(* Logix 5000 AddOnInstructionDefinition export HI6200_Faceplate_IT_AOI; software revision 30.00; part 2 of 2 *)
(* tags used below, declared in another part *)
   Inp_hi6200 : _0102:Hardy6200Series_F6857DC7:I:0;
   Out_hi6200 : _0102:Hardy6200Series_52E4DDE0:O:0;
   IT_Status : DINT;   // Integrated Technician status indication
   pm_49C1 : REAL;   // WAVERSAVER VAR ch 1
   pm_49C2 : REAL;   // WAVERSAVER VAR ch 2
   pm_49C3 : REAL;   // WAVERSAVER VAR ch 3
   pm_49C8 : REAL;   // WAVERSAVER VAR ref 1
   pm_49C4 : REAL;   // WAVERSAVER VAR ch 4
   pm_49C5 : REAL;   // WAVERSAVER VAR ch 5
   pm_49C6 : REAL;   // WAVERSAVER VAR ch 6
   pm_49C7 : REAL;   // WAVERSAVER VAR ch 7
   pm_49C9 : REAL;   // WAVERSAVER VAR ref 2
   pm_49D0 : DINT;   // RAW VAR results ch 0
   pm_49D1 : DINT;   // RAW VAR results ch 1
   pm_49D2 : DINT;   // RAW VAR results ch 2
   pm_49D3 : DINT;   // RAW VAR results ch 3
   pm_49D8 : DINT;   // RAW VAR results ref 1
   pm_49D4 : DINT;   // RAW VAR results ch 4
   pm_49D5 : DINT;   // RAW VAR results ch 5
   pm_49D6 : DINT;   // RAW VAR results ch 6
   pm_49D7 : DINT;   // RAW VAR results ch 7
   pm_49D9 : DINT;   // RAW VAR results ref 2
   pm_49E0 : DINT;   // WAVERSAVER VAR results ch 0
   pm_49E1 : DINT;   // WAVERSAVER VAR results ch 1
   pm_49E2 : DINT;   // WAVERSAVER VAR results ch 2
   pm_49E3 : DINT;   // WAVERSAVER VAR results ch 3
   pm_49E8 : DINT;   // WAVERSAVER VAR results ref 1
   pm_49E4 : DINT;   // WAVERSAVER VAR results ch 4
   pm_49E5 : DINT;   // WAVERSAVER VAR results ch 5
   pm_49E6 : DINT;   // WAVERSAVER VAR results ch 6
   pm_49E7 : DINT;   // WAVERSAVER VAR results ch 7
   pm_49E9 : DINT;   // WAVERSAVER VAR results ref 2
   rd_rtz : INT;   // return to zero status
   pm_49F0 : DINT;   // RTZ ch 0
   pm_49F1 : DINT;   // RTZ ch 1
   pm_49F2 : DINT;   // RTZ ch 2
   pm_49F3 : DINT;   // RTZ ch 3
   pm_49F4 : DINT;   // RTZ ch 4
   pm_49F5 : DINT;   // RTZ ch 5
   pm_49F6 : DINT;   // RTZ ch 6
   pm_49F7 : DINT;   // RTZ ch 7
   pm_498C : DINT;   // RTZ combined
   IT_running_status : DINT;   // running/status indication
   rd_ws_var : INT;   // trigger to read WAVERSAVER variation
   rd_raw_rst : INT;   // trigger to read raw variation results
   rd_ws_rst : INT;   // trigger to read WAVERSAVER results
   rd_jbox_2_too : BOOL;   // Process control bit
   delay_clear : TIMER;   // time delay to copy value
   read_delay_29 : TIMER;   // time delay to copy value
   read_delay_30 : TIMER;   // time delay to copy value
   read_delay_31 : TIMER;   // time delay to copy value
   read_delay_32 : TIMER;   // time delay to copy value
   read_delay_33 : TIMER;   // time delay to copy value
   read_delay_34 : TIMER;   // time delay to copy value
   read_delay_35 : TIMER;   // time delay to copy value
   read_delay_36 : TIMER;   // time delay to copy value
   read_delay_37 : TIMER;   // time delay to copy value
   read_delay_38 : TIMER;   // time delay to copy value
   read_delay_39 : TIMER;   // time delay to copy value
   read_delay_40 : TIMER;   // time delay to copy value
   read_delay_41 : TIMER;   // time delay to copy value
   read_delay_42 : TIMER;   // time delay to copy value
   read_delay_43 : TIMER;   // time delay to copy value
   read_delay_44 : TIMER;   // time delay to copy value
   read_delay_45 : TIMER;   // time delay to copy value
   read_delay_46 : TIMER;   // time delay to copy value
   read_delay_47 : TIMER;   // time delay to copy value
   read_delay_48 : TIMER;   // time delay to copy value
   read_delay_49 : TIMER;   // time delay to copy value
   read_delay_50 : TIMER;   // time delay to copy value
   read_delay_51 : TIMER;   // time delay to copy value
   read_delay_52 : TIMER;   // time delay to copy value
   read_delay_53 : TIMER;   // time delay to copy value
   read_delay_54 : TIMER;   // time delay to copy value
   read_delay_55 : TIMER;   // time delay to copy value
   read_delay_56 : TIMER;   // time delay to copy value
   read_delay_57 : TIMER;   // time delay to copy value
   read_delay_58 : TIMER;   // time delay to copy value
   read_delay_59 : TIMER;   // time delay to copy value
   read_delay_60 : TIMER;   // time delay to copy value
   read_delay_61 : TIMER;   // time delay to copy value
   read_delay_62 : TIMER;   // time delay to copy value
   read_delay_63 : TIMER;   // time delay to copy value
   read_delay_64 : TIMER;   // time delay to copy value
   read_delay_65 : TIMER;   // time delay to copy value
   read_delay_66 : TIMER;   // time delay to copy value
   read_delay_67 : TIMER;   // time delay to copy value
   clear_status : BOOL;   // process control bit
(* HI6200_Faceplate_IT_AOI, continued *)

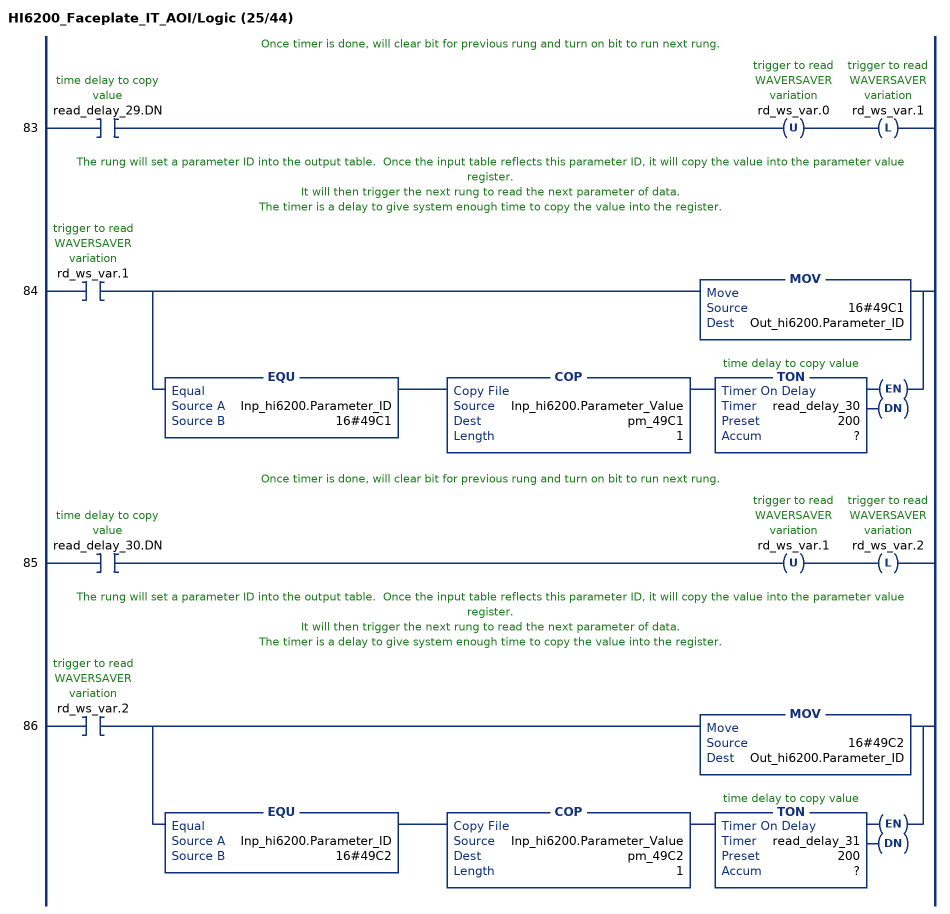
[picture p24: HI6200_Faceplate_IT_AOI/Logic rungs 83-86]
   // Once timer is done, will clear bit for previous rung and turn on bit to run next rung.
   83: XIC(read_delay_29.DN)OTU(rd_ws_var.0)OTL(rd_ws_var.1);
   // The rung will set a parameter ID into the output table.  Once the input table reflects this parameter ID, it will copy the value into the parameter value register.
   // It will then trigger the next rung to read the next parameter of data.
   // The timer is a delay to give system enough time to copy the value into the register.
   84: XIC(rd_ws_var.1)[MOV(16#49C1,Out_hi6200.Parameter_ID) ,EQU(Inp_hi6200.Parameter_ID,16#49C1) COP(Inp_hi6200.Parameter_Value,pm_49C1,1) TON(read_delay_30,?,?) ];
   // Once timer is done, will clear bit for previous rung and turn on bit to run next rung.
   85: XIC(read_delay_30.DN)OTU(rd_ws_var.1)OTL(rd_ws_var.2);
   // The rung will set a parameter ID into the output table.  Once the input table reflects this parameter ID, it will copy the value into the parameter value register.
   // It will then trigger the next rung to read the next parameter of data.
   // The timer is a delay to give system enough time to copy the value into the register.
   86: XIC(rd_ws_var.2)[MOV(16#49C2,Out_hi6200.Parameter_ID) ,EQU(Inp_hi6200.Parameter_ID,16#49C2) COP(Inp_hi6200.Parameter_Value,pm_49C2,1) TON(read_delay_31,?,?) ];
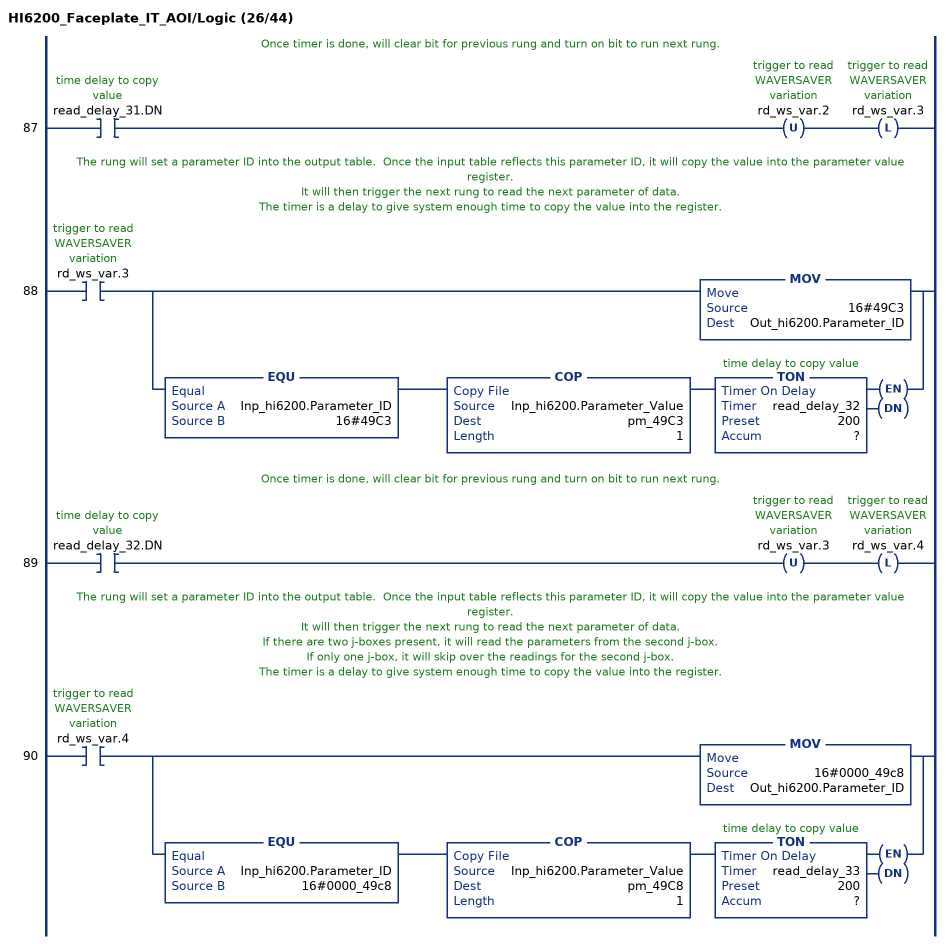
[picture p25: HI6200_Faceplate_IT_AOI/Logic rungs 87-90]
   // Once timer is done, will clear bit for previous rung and turn on bit to run next rung.
   87: XIC(read_delay_31.DN)OTU(rd_ws_var.2)OTL(rd_ws_var.3);
   // The rung will set a parameter ID into the output table.  Once the input table reflects this parameter ID, it will copy the value into the parameter value register.
   // It will then trigger the next rung to read the next parameter of data.
   // The timer is a delay to give system enough time to copy the value into the register.
   88: XIC(rd_ws_var.3)[MOV(16#49C3,Out_hi6200.Parameter_ID) ,EQU(Inp_hi6200.Parameter_ID,16#49C3) COP(Inp_hi6200.Parameter_Value,pm_49C3,1) TON(read_delay_32,?,?) ];
   // Once timer is done, will clear bit for previous rung and turn on bit to run next rung.
   89: XIC(read_delay_32.DN)OTU(rd_ws_var.3)OTL(rd_ws_var.4);
   // The rung will set a parameter ID into the output table.  Once the input table reflects this parameter ID, it will copy the value into the parameter value register.
   // It will then trigger the next rung to read the next parameter of data.
   // If there are two j-boxes present, it will read the parameters from the second j-box.
   // If only one j-box, it will skip over the readings for the second j-box.
   // The timer is a delay to give system enough time to copy the value into the register.
   90: XIC(rd_ws_var.4)[MOV(16#0000_49c8,Out_hi6200.Parameter_ID) ,EQU(Inp_hi6200.Parameter_ID,16#0000_49c8) COP(Inp_hi6200.Parameter_Value,pm_49C8,1) TON(read_delay_33,?,?) ];
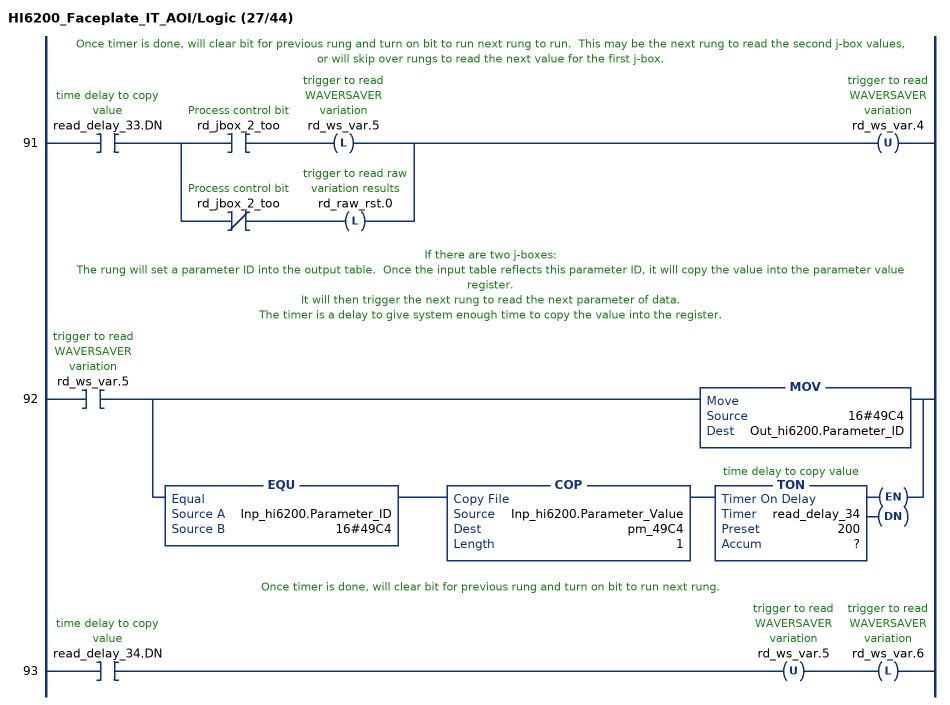
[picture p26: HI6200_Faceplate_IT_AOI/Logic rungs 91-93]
   // Once timer is done, will clear bit for previous rung and turn on bit to run next rung to run.  This may be the next rung to read the second j-box values, or will skip over rungs to read the next value for the first j-box.
   91: XIC(read_delay_33.DN)[XIC(rd_jbox_2_too) OTL(rd_ws_var.5) ,XIO(rd_jbox_2_too) OTL(rd_raw_rst.0) ]OTU(rd_ws_var.4);
   // If there are two j-boxes:
   // The rung will set a parameter ID into the output table.  Once the input table reflects this parameter ID, it will copy the value into the parameter value register.
   // It will then trigger the next rung to read the next parameter of data.
   // The timer is a delay to give system enough time to copy the value into the register.
   92: XIC(rd_ws_var.5)[MOV(16#49C4,Out_hi6200.Parameter_ID) ,EQU(Inp_hi6200.Parameter_ID,16#49C4) COP(Inp_hi6200.Parameter_Value,pm_49C4,1) TON(read_delay_34,?,?) ];
   // Once timer is done, will clear bit for previous rung and turn on bit to run next rung.
   93: XIC(read_delay_34.DN)OTU(rd_ws_var.5)OTL(rd_ws_var.6);
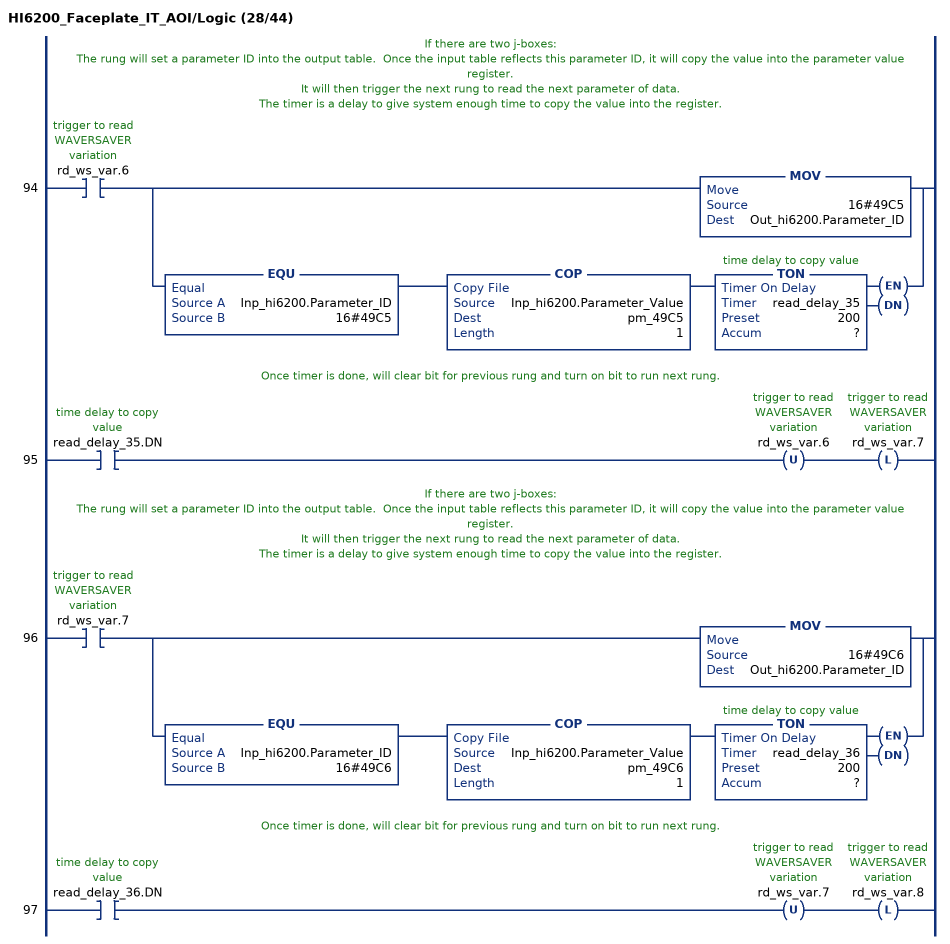
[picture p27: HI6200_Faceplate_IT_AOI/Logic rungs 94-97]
   // If there are two j-boxes:
   // The rung will set a parameter ID into the output table.  Once the input table reflects this parameter ID, it will copy the value into the parameter value register.
   // It will then trigger the next rung to read the next parameter of data.
   // The timer is a delay to give system enough time to copy the value into the register.
   94: XIC(rd_ws_var.6)[MOV(16#49C5,Out_hi6200.Parameter_ID) ,EQU(Inp_hi6200.Parameter_ID,16#49C5) COP(Inp_hi6200.Parameter_Value,pm_49C5,1) TON(read_delay_35,?,?) ];
   // Once timer is done, will clear bit for previous rung and turn on bit to run next rung.
   95: XIC(read_delay_35.DN)OTU(rd_ws_var.6)OTL(rd_ws_var.7);
   // If there are two j-boxes:
   // The rung will set a parameter ID into the output table.  Once the input table reflects this parameter ID, it will copy the value into the parameter value register.
   // It will then trigger the next rung to read the next parameter of data.
   // The timer is a delay to give system enough time to copy the value into the register.
   96: XIC(rd_ws_var.7)[MOV(16#49C6,Out_hi6200.Parameter_ID) ,EQU(Inp_hi6200.Parameter_ID,16#49C6) COP(Inp_hi6200.Parameter_Value,pm_49C6,1) TON(read_delay_36,?,?) ];
   // Once timer is done, will clear bit for previous rung and turn on bit to run next rung.
   97: XIC(read_delay_36.DN)OTU(rd_ws_var.7)OTL(rd_ws_var.8);
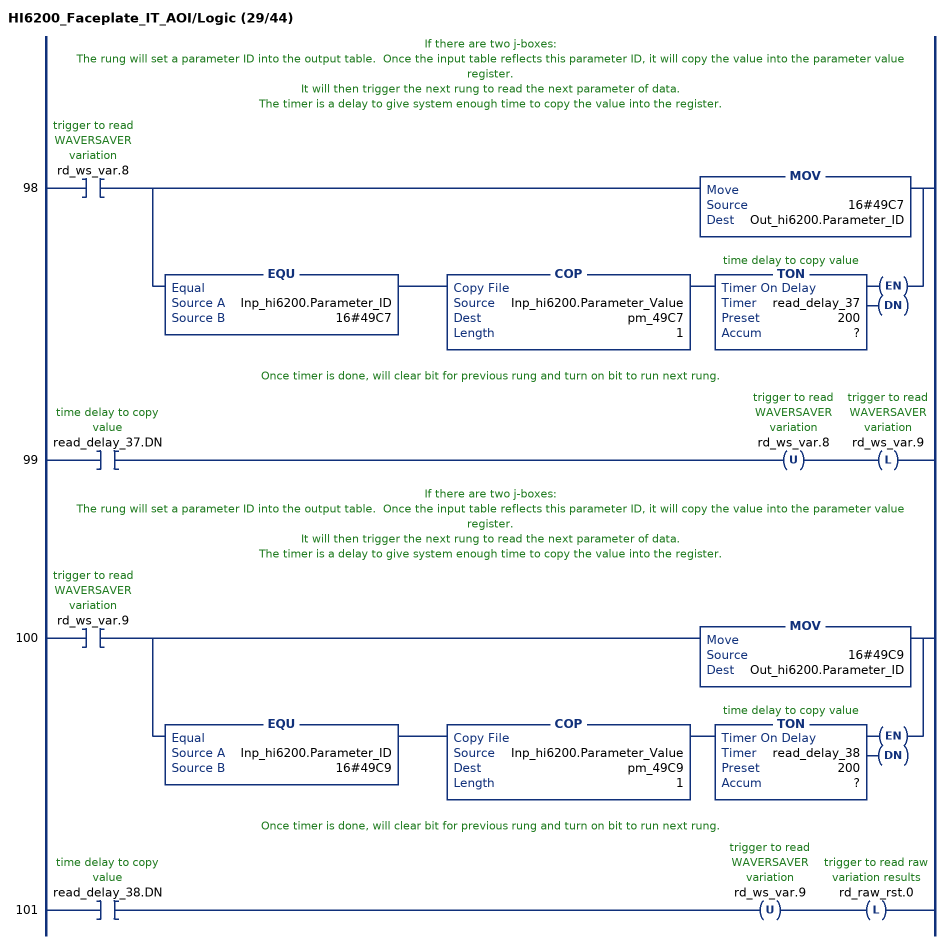
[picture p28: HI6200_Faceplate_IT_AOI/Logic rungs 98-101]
   // If there are two j-boxes:
   // The rung will set a parameter ID into the output table.  Once the input table reflects this parameter ID, it will copy the value into the parameter value register.
   // It will then trigger the next rung to read the next parameter of data.
   // The timer is a delay to give system enough time to copy the value into the register.
   98: XIC(rd_ws_var.8)[MOV(16#49C7,Out_hi6200.Parameter_ID) ,EQU(Inp_hi6200.Parameter_ID,16#49C7) COP(Inp_hi6200.Parameter_Value,pm_49C7,1) TON(read_delay_37,?,?) ];
   // Once timer is done, will clear bit for previous rung and turn on bit to run next rung.
   99: XIC(read_delay_37.DN)OTU(rd_ws_var.8)OTL(rd_ws_var.9);
   // If there are two j-boxes:
   // The rung will set a parameter ID into the output table.  Once the input table reflects this parameter ID, it will copy the value into the parameter value register.
   // It will then trigger the next rung to read the next parameter of data.
   // The timer is a delay to give system enough time to copy the value into the register.
   100: XIC(rd_ws_var.9)[MOV(16#49C9,Out_hi6200.Parameter_ID) ,EQU(Inp_hi6200.Parameter_ID,16#49C9) COP(Inp_hi6200.Parameter_Value,pm_49C9,1) TON(read_delay_38,?,?) ];
   // Once timer is done, will clear bit for previous rung and turn on bit to run next rung.
   101: XIC(read_delay_38.DN)OTU(rd_ws_var.9)OTL(rd_raw_rst.0);
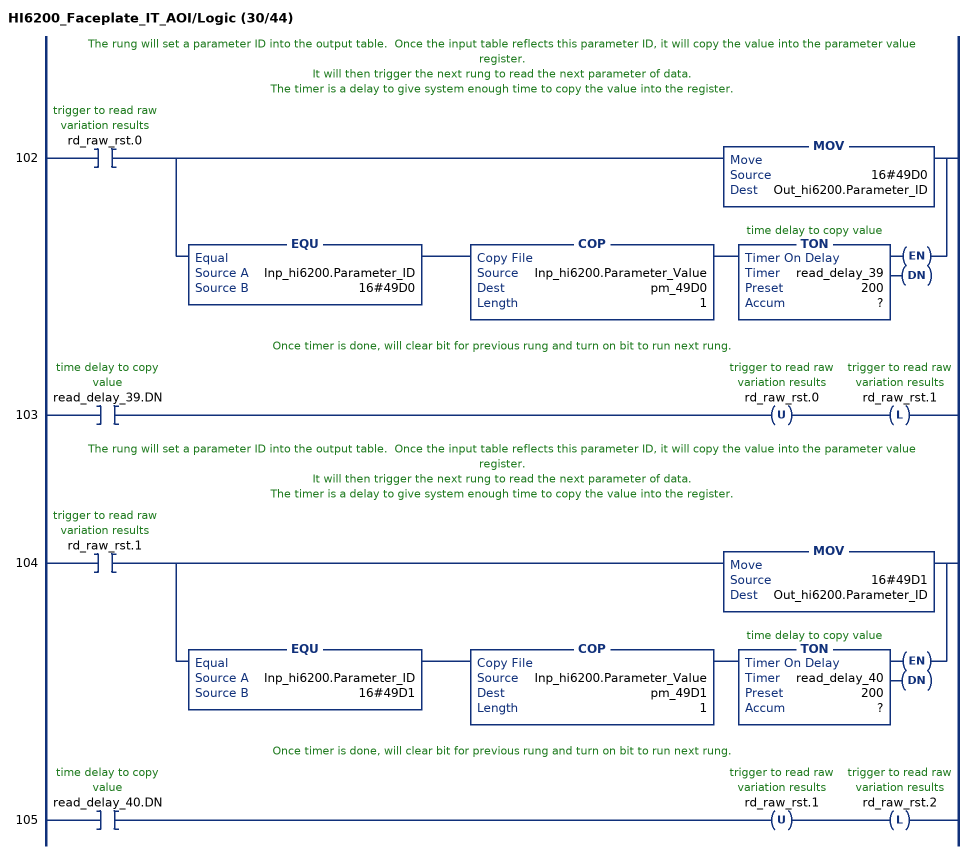
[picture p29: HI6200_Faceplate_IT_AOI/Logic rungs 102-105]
   // The rung will set a parameter ID into the output table.  Once the input table reflects this parameter ID, it will copy the value into the parameter value register.
   // It will then trigger the next rung to read the next parameter of data.
   // The timer is a delay to give system enough time to copy the value into the register.
   102: XIC(rd_raw_rst.0)[MOV(16#49D0,Out_hi6200.Parameter_ID) ,EQU(Inp_hi6200.Parameter_ID,16#49D0) COP(Inp_hi6200.Parameter_Value,pm_49D0,1) TON(read_delay_39,?,?) ];
   // Once timer is done, will clear bit for previous rung and turn on bit to run next rung.
   103: XIC(read_delay_39.DN)OTU(rd_raw_rst.0)OTL(rd_raw_rst.1);
   // The rung will set a parameter ID into the output table.  Once the input table reflects this parameter ID, it will copy the value into the parameter value register.
   // It will then trigger the next rung to read the next parameter of data.
   // The timer is a delay to give system enough time to copy the value into the register.
   104: XIC(rd_raw_rst.1)[MOV(16#49D1,Out_hi6200.Parameter_ID) ,EQU(Inp_hi6200.Parameter_ID,16#49D1) COP(Inp_hi6200.Parameter_Value,pm_49D1,1) TON(read_delay_40,?,?) ];
   // Once timer is done, will clear bit for previous rung and turn on bit to run next rung.
   105: XIC(read_delay_40.DN)OTU(rd_raw_rst.1)OTL(rd_raw_rst.2);
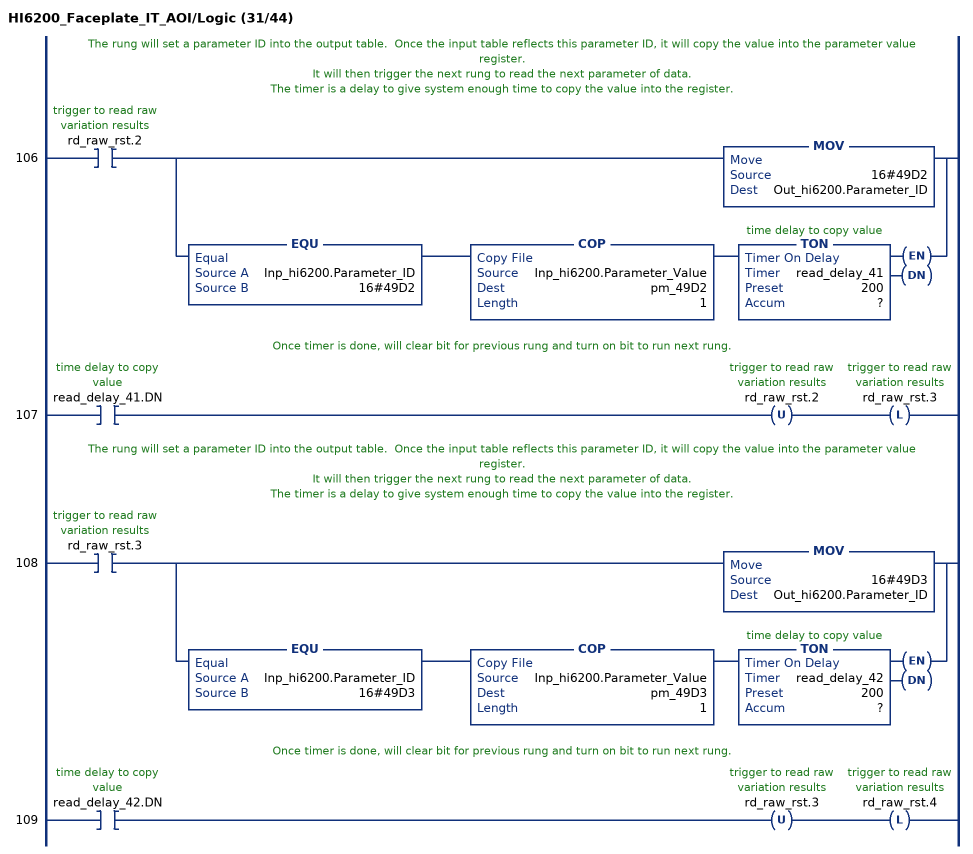
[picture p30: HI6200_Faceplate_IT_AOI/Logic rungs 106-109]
   // The rung will set a parameter ID into the output table.  Once the input table reflects this parameter ID, it will copy the value into the parameter value register.
   // It will then trigger the next rung to read the next parameter of data.
   // The timer is a delay to give system enough time to copy the value into the register.
   106: XIC(rd_raw_rst.2)[MOV(16#49D2,Out_hi6200.Parameter_ID) ,EQU(Inp_hi6200.Parameter_ID,16#49D2) COP(Inp_hi6200.Parameter_Value,pm_49D2,1) TON(read_delay_41,?,?) ];
   // Once timer is done, will clear bit for previous rung and turn on bit to run next rung.
   107: XIC(read_delay_41.DN)OTU(rd_raw_rst.2)OTL(rd_raw_rst.3);
   // The rung will set a parameter ID into the output table.  Once the input table reflects this parameter ID, it will copy the value into the parameter value register.
   // It will then trigger the next rung to read the next parameter of data.
   // The timer is a delay to give system enough time to copy the value into the register.
   108: XIC(rd_raw_rst.3)[MOV(16#49D3,Out_hi6200.Parameter_ID) ,EQU(Inp_hi6200.Parameter_ID,16#49D3) COP(Inp_hi6200.Parameter_Value,pm_49D3,1) TON(read_delay_42,?,?) ];
   // Once timer is done, will clear bit for previous rung and turn on bit to run next rung.
   109: XIC(read_delay_42.DN)OTU(rd_raw_rst.3)OTL(rd_raw_rst.4);
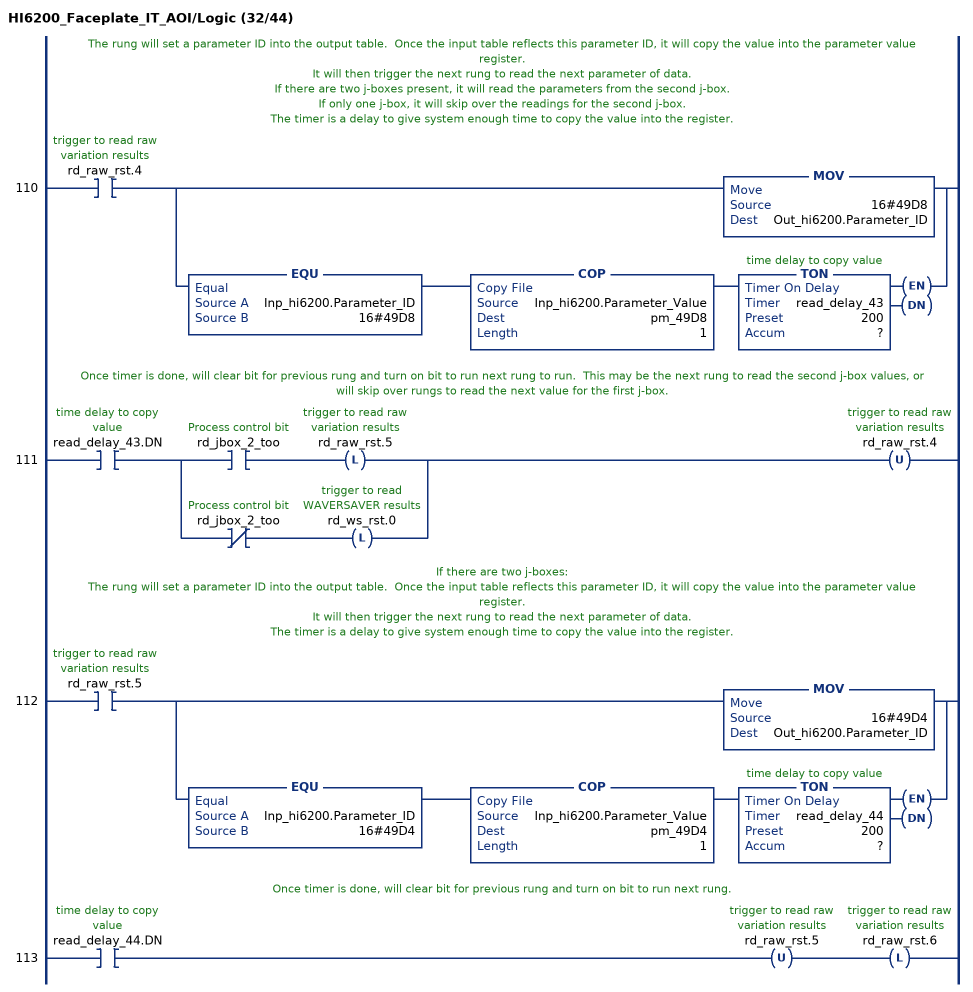
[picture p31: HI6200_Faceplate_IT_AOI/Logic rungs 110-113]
   // The rung will set a parameter ID into the output table.  Once the input table reflects this parameter ID, it will copy the value into the parameter value register.
   // It will then trigger the next rung to read the next parameter of data.
   // If there are two j-boxes present, it will read the parameters from the second j-box.
   // If only one j-box, it will skip over the readings for the second j-box.
   // The timer is a delay to give system enough time to copy the value into the register.
   110: XIC(rd_raw_rst.4)[MOV(16#49D8,Out_hi6200.Parameter_ID) ,EQU(Inp_hi6200.Parameter_ID,16#49D8) COP(Inp_hi6200.Parameter_Value,pm_49D8,1) TON(read_delay_43,?,?) ];
   // Once timer is done, will clear bit for previous rung and turn on bit to run next rung to run.  This may be the next rung to read the second j-box values, or will skip over rungs to read the next value for the first j-box.
   111: XIC(read_delay_43.DN)[XIC(rd_jbox_2_too) OTL(rd_raw_rst.5) ,XIO(rd_jbox_2_too) OTL(rd_ws_rst.0) ]OTU(rd_raw_rst.4);
   // If there are two j-boxes:
   // The rung will set a parameter ID into the output table.  Once the input table reflects this parameter ID, it will copy the value into the parameter value register.
   // It will then trigger the next rung to read the next parameter of data.
   // The timer is a delay to give system enough time to copy the value into the register.
   112: XIC(rd_raw_rst.5)[MOV(16#49D4,Out_hi6200.Parameter_ID) ,EQU(Inp_hi6200.Parameter_ID,16#49D4) COP(Inp_hi6200.Parameter_Value,pm_49D4,1) TON(read_delay_44,?,?) ];
   // Once timer is done, will clear bit for previous rung and turn on bit to run next rung.
   113: XIC(read_delay_44.DN)OTU(rd_raw_rst.5)OTL(rd_raw_rst.6);
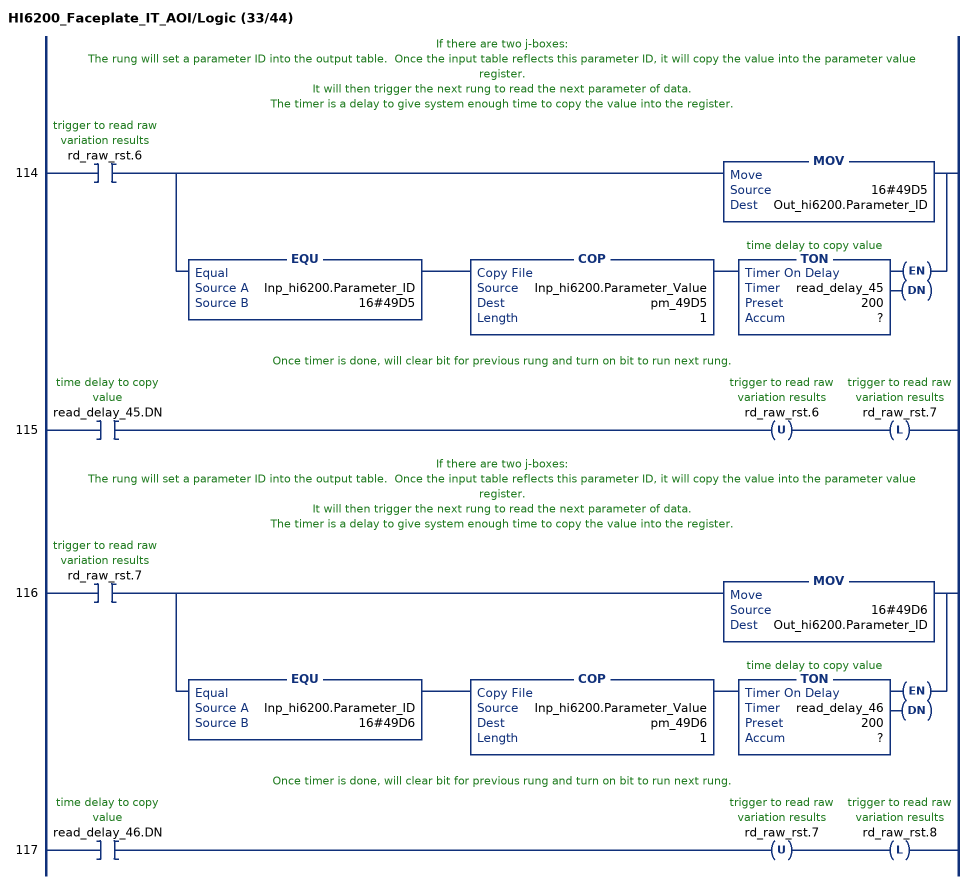
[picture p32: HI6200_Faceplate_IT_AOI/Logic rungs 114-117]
   // If there are two j-boxes:
   // The rung will set a parameter ID into the output table.  Once the input table reflects this parameter ID, it will copy the value into the parameter value register.
   // It will then trigger the next rung to read the next parameter of data.
   // The timer is a delay to give system enough time to copy the value into the register.
   114: XIC(rd_raw_rst.6)[MOV(16#49D5,Out_hi6200.Parameter_ID) ,EQU(Inp_hi6200.Parameter_ID,16#49D5) COP(Inp_hi6200.Parameter_Value,pm_49D5,1) TON(read_delay_45,?,?) ];
   // Once timer is done, will clear bit for previous rung and turn on bit to run next rung.
   115: XIC(read_delay_45.DN)OTU(rd_raw_rst.6)OTL(rd_raw_rst.7);
   // If there are two j-boxes:
   // The rung will set a parameter ID into the output table.  Once the input table reflects this parameter ID, it will copy the value into the parameter value register.
   // It will then trigger the next rung to read the next parameter of data.
   // The timer is a delay to give system enough time to copy the value into the register.
   116: XIC(rd_raw_rst.7)[MOV(16#49D6,Out_hi6200.Parameter_ID) ,EQU(Inp_hi6200.Parameter_ID,16#49D6) COP(Inp_hi6200.Parameter_Value,pm_49D6,1) TON(read_delay_46,?,?) ];
   // Once timer is done, will clear bit for previous rung and turn on bit to run next rung.
   117: XIC(read_delay_46.DN)OTU(rd_raw_rst.7)OTL(rd_raw_rst.8);
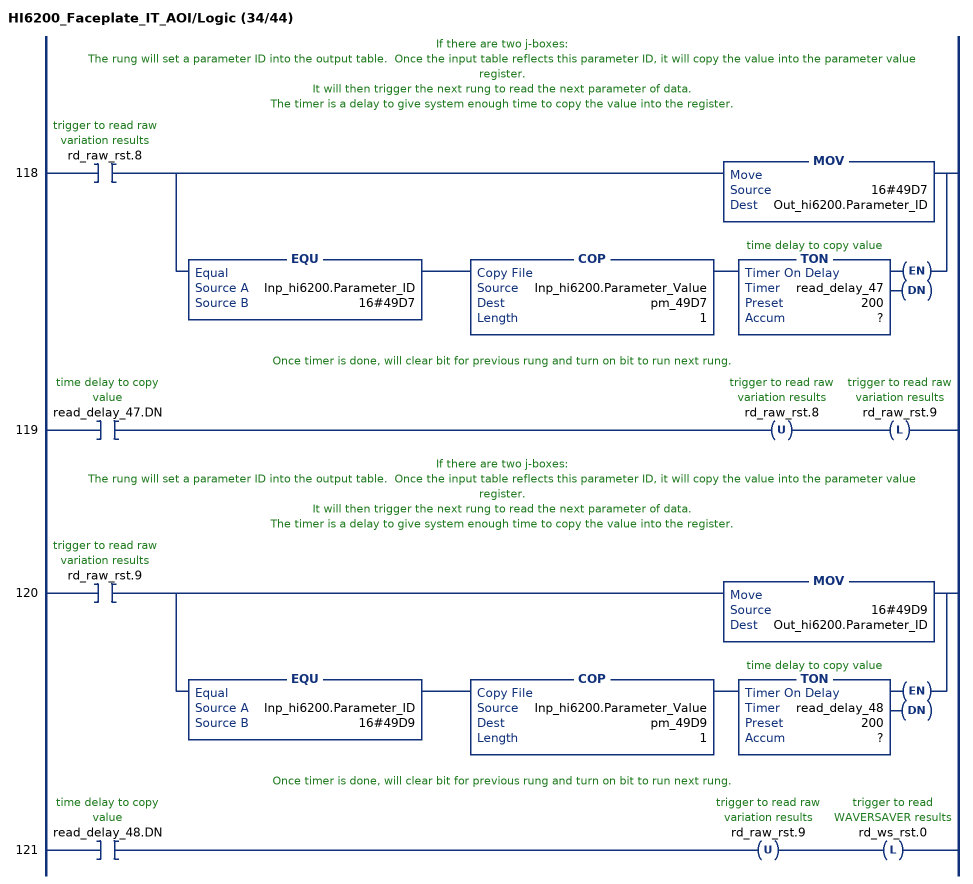
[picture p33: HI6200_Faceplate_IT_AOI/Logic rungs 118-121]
   // If there are two j-boxes:
   // The rung will set a parameter ID into the output table.  Once the input table reflects this parameter ID, it will copy the value into the parameter value register.
   // It will then trigger the next rung to read the next parameter of data.
   // The timer is a delay to give system enough time to copy the value into the register.
   118: XIC(rd_raw_rst.8)[MOV(16#49D7,Out_hi6200.Parameter_ID) ,EQU(Inp_hi6200.Parameter_ID,16#49D7) COP(Inp_hi6200.Parameter_Value,pm_49D7,1) TON(read_delay_47,?,?) ];
   // Once timer is done, will clear bit for previous rung and turn on bit to run next rung.
   119: XIC(read_delay_47.DN)OTU(rd_raw_rst.8)OTL(rd_raw_rst.9);
   // If there are two j-boxes:
   // The rung will set a parameter ID into the output table.  Once the input table reflects this parameter ID, it will copy the value into the parameter value register.
   // It will then trigger the next rung to read the next parameter of data.
   // The timer is a delay to give system enough time to copy the value into the register.
   120: XIC(rd_raw_rst.9)[MOV(16#49D9,Out_hi6200.Parameter_ID) ,EQU(Inp_hi6200.Parameter_ID,16#49D9) COP(Inp_hi6200.Parameter_Value,pm_49D9,1) TON(read_delay_48,?,?) ];
   // Once timer is done, will clear bit for previous rung and turn on bit to run next rung.
   121: XIC(read_delay_48.DN)OTU(rd_raw_rst.9)OTL(rd_ws_rst.0);
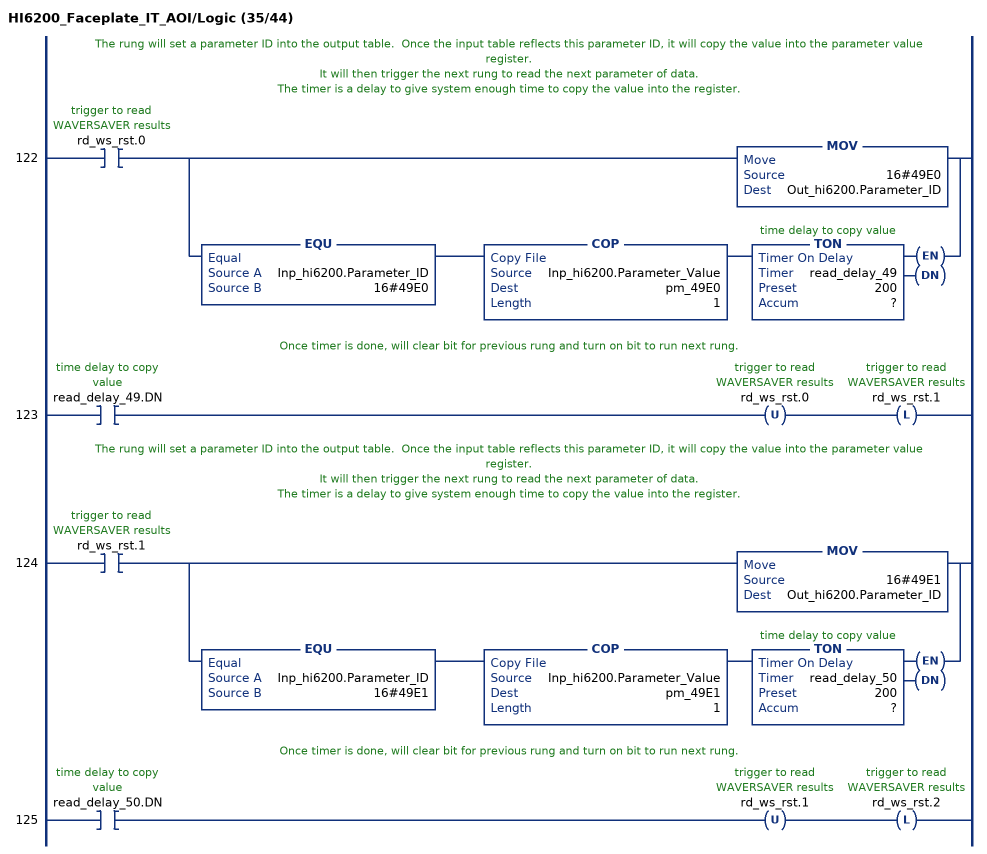
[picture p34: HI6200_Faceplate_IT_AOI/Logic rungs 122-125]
   // The rung will set a parameter ID into the output table.  Once the input table reflects this parameter ID, it will copy the value into the parameter value register.
   // It will then trigger the next rung to read the next parameter of data.
   // The timer is a delay to give system enough time to copy the value into the register.
   122: XIC(rd_ws_rst.0)[MOV(16#49E0,Out_hi6200.Parameter_ID) ,EQU(Inp_hi6200.Parameter_ID,16#49E0) COP(Inp_hi6200.Parameter_Value,pm_49E0,1) TON(read_delay_49,?,?) ];
   // Once timer is done, will clear bit for previous rung and turn on bit to run next rung.
   123: XIC(read_delay_49.DN)OTU(rd_ws_rst.0)OTL(rd_ws_rst.1);
   // The rung will set a parameter ID into the output table.  Once the input table reflects this parameter ID, it will copy the value into the parameter value register.
   // It will then trigger the next rung to read the next parameter of data.
   // The timer is a delay to give system enough time to copy the value into the register.
   124: XIC(rd_ws_rst.1)[MOV(16#49E1,Out_hi6200.Parameter_ID) ,EQU(Inp_hi6200.Parameter_ID,16#49E1) COP(Inp_hi6200.Parameter_Value,pm_49E1,1) TON(read_delay_50,?,?) ];
   // Once timer is done, will clear bit for previous rung and turn on bit to run next rung.
   125: XIC(read_delay_50.DN)OTU(rd_ws_rst.1)OTL(rd_ws_rst.2);
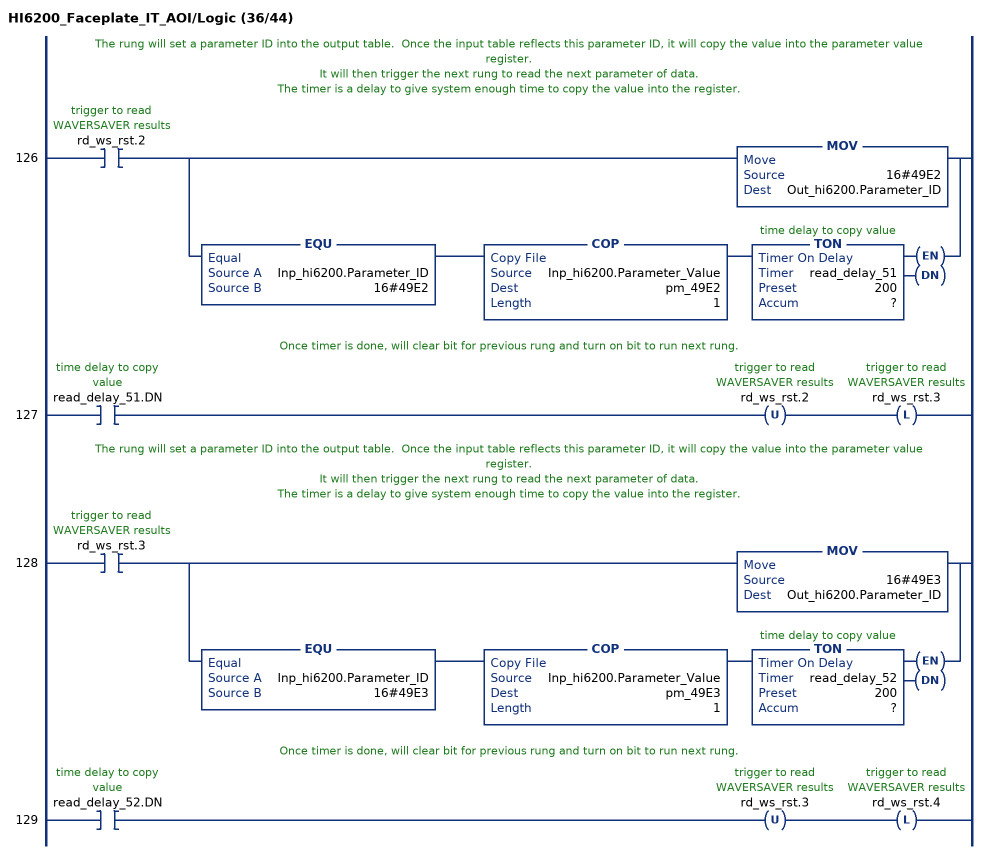
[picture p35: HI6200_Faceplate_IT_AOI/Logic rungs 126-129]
   // The rung will set a parameter ID into the output table.  Once the input table reflects this parameter ID, it will copy the value into the parameter value register.
   // It will then trigger the next rung to read the next parameter of data.
   // The timer is a delay to give system enough time to copy the value into the register.
   126: XIC(rd_ws_rst.2)[MOV(16#49E2,Out_hi6200.Parameter_ID) ,EQU(Inp_hi6200.Parameter_ID,16#49E2) COP(Inp_hi6200.Parameter_Value,pm_49E2,1) TON(read_delay_51,?,?) ];
   // Once timer is done, will clear bit for previous rung and turn on bit to run next rung.
   127: XIC(read_delay_51.DN)OTU(rd_ws_rst.2)OTL(rd_ws_rst.3);
   // The rung will set a parameter ID into the output table.  Once the input table reflects this parameter ID, it will copy the value into the parameter value register.
   // It will then trigger the next rung to read the next parameter of data.
   // The timer is a delay to give system enough time to copy the value into the register.
   128: XIC(rd_ws_rst.3)[MOV(16#49E3,Out_hi6200.Parameter_ID) ,EQU(Inp_hi6200.Parameter_ID,16#49E3) COP(Inp_hi6200.Parameter_Value,pm_49E3,1) TON(read_delay_52,?,?) ];
   // Once timer is done, will clear bit for previous rung and turn on bit to run next rung.
   129: XIC(read_delay_52.DN)OTU(rd_ws_rst.3)OTL(rd_ws_rst.4);
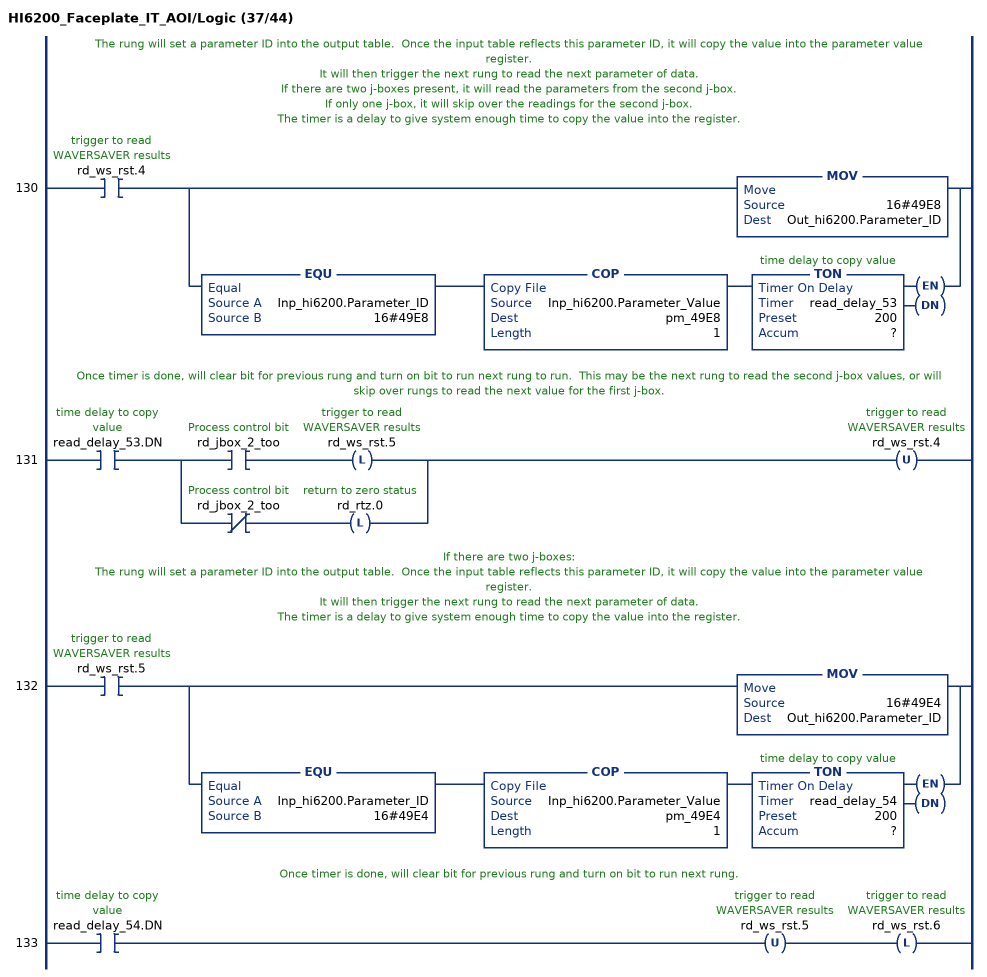
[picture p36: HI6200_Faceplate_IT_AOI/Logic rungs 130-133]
   // The rung will set a parameter ID into the output table.  Once the input table reflects this parameter ID, it will copy the value into the parameter value register.
   // It will then trigger the next rung to read the next parameter of data.
   // If there are two j-boxes present, it will read the parameters from the second j-box.
   // If only one j-box, it will skip over the readings for the second j-box.
   // The timer is a delay to give system enough time to copy the value into the register.
   130: XIC(rd_ws_rst.4)[MOV(16#49E8,Out_hi6200.Parameter_ID) ,EQU(Inp_hi6200.Parameter_ID,16#49E8) COP(Inp_hi6200.Parameter_Value,pm_49E8,1) TON(read_delay_53,?,?) ];
   // Once timer is done, will clear bit for previous rung and turn on bit to run next rung to run.  This may be the next rung to read the second j-box values, or will skip over rungs to read the next value for the first j-box.
   131: XIC(read_delay_53.DN)[XIC(rd_jbox_2_too) OTL(rd_ws_rst.5) ,XIO(rd_jbox_2_too) OTL(rd_rtz.0) ]OTU(rd_ws_rst.4);
   // If there are two j-boxes:
   // The rung will set a parameter ID into the output table.  Once the input table reflects this parameter ID, it will copy the value into the parameter value register.
   // It will then trigger the next rung to read the next parameter of data.
   // The timer is a delay to give system enough time to copy the value into the register.
   132: XIC(rd_ws_rst.5)[MOV(16#49E4,Out_hi6200.Parameter_ID) ,EQU(Inp_hi6200.Parameter_ID,16#49E4) COP(Inp_hi6200.Parameter_Value,pm_49E4,1) TON(read_delay_54,?,?) ];
   // Once timer is done, will clear bit for previous rung and turn on bit to run next rung.
   133: XIC(read_delay_54.DN)OTU(rd_ws_rst.5)OTL(rd_ws_rst.6);
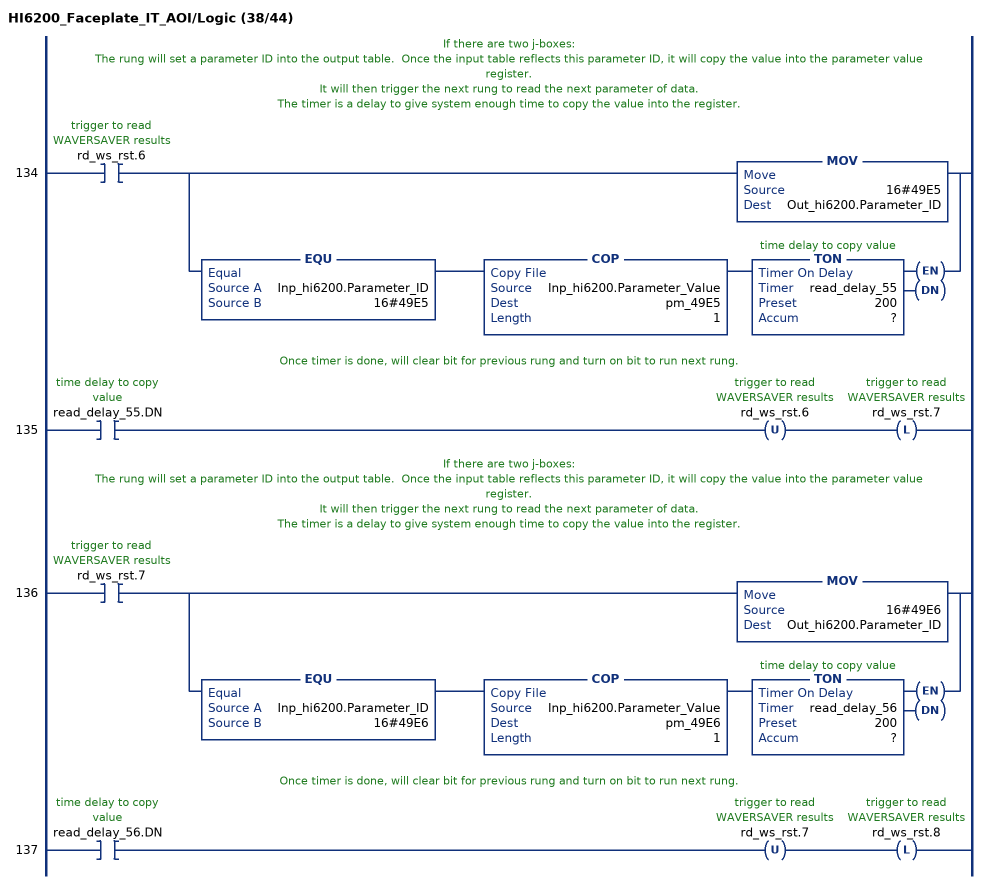
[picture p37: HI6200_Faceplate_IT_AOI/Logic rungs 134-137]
   // If there are two j-boxes:
   // The rung will set a parameter ID into the output table.  Once the input table reflects this parameter ID, it will copy the value into the parameter value register.
   // It will then trigger the next rung to read the next parameter of data.
   // The timer is a delay to give system enough time to copy the value into the register.
   134: XIC(rd_ws_rst.6)[MOV(16#49E5,Out_hi6200.Parameter_ID) ,EQU(Inp_hi6200.Parameter_ID,16#49E5) COP(Inp_hi6200.Parameter_Value,pm_49E5,1) TON(read_delay_55,?,?) ];
   // Once timer is done, will clear bit for previous rung and turn on bit to run next rung.
   135: XIC(read_delay_55.DN)OTU(rd_ws_rst.6)OTL(rd_ws_rst.7);
   // If there are two j-boxes:
   // The rung will set a parameter ID into the output table.  Once the input table reflects this parameter ID, it will copy the value into the parameter value register.
   // It will then trigger the next rung to read the next parameter of data.
   // The timer is a delay to give system enough time to copy the value into the register.
   136: XIC(rd_ws_rst.7)[MOV(16#49E6,Out_hi6200.Parameter_ID) ,EQU(Inp_hi6200.Parameter_ID,16#49E6) COP(Inp_hi6200.Parameter_Value,pm_49E6,1) TON(read_delay_56,?,?) ];
   // Once timer is done, will clear bit for previous rung and turn on bit to run next rung.
   137: XIC(read_delay_56.DN)OTU(rd_ws_rst.7)OTL(rd_ws_rst.8);
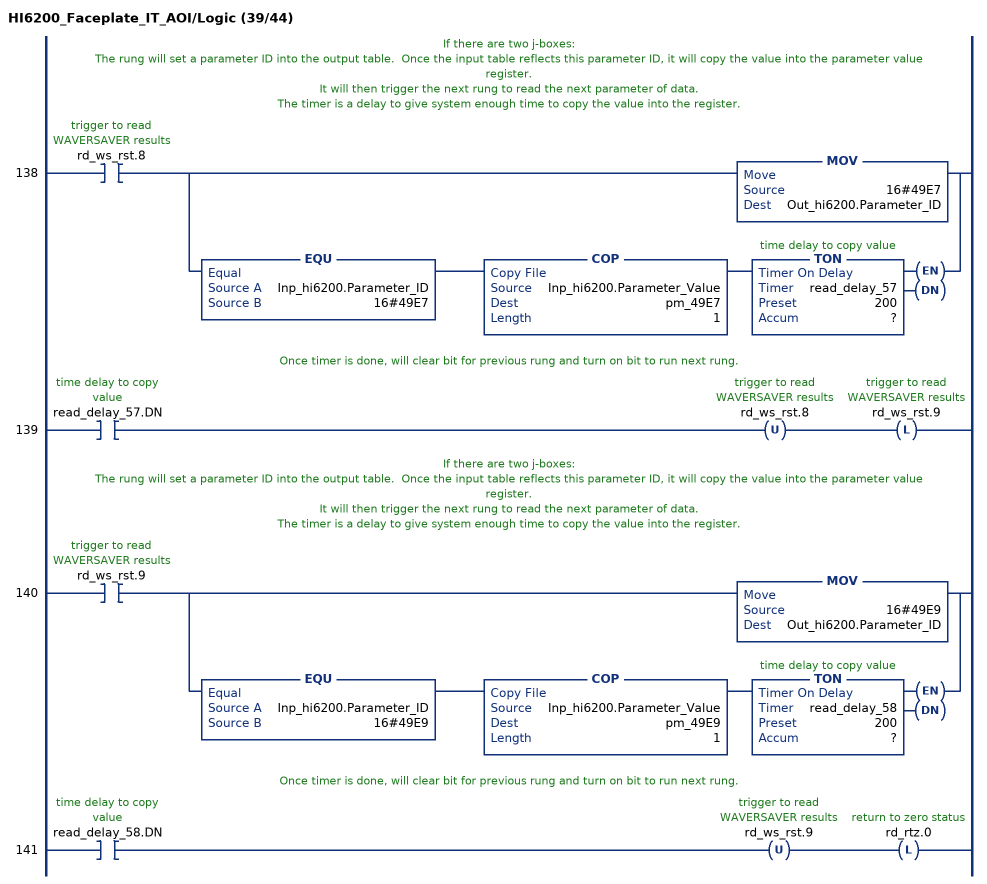
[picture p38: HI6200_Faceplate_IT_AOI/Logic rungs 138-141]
   // If there are two j-boxes:
   // The rung will set a parameter ID into the output table.  Once the input table reflects this parameter ID, it will copy the value into the parameter value register.
   // It will then trigger the next rung to read the next parameter of data.
   // The timer is a delay to give system enough time to copy the value into the register.
   138: XIC(rd_ws_rst.8)[MOV(16#49E7,Out_hi6200.Parameter_ID) ,EQU(Inp_hi6200.Parameter_ID,16#49E7) COP(Inp_hi6200.Parameter_Value,pm_49E7,1) TON(read_delay_57,?,?) ];
   // Once timer is done, will clear bit for previous rung and turn on bit to run next rung.
   139: XIC(read_delay_57.DN)OTU(rd_ws_rst.8)OTL(rd_ws_rst.9);
   // If there are two j-boxes:
   // The rung will set a parameter ID into the output table.  Once the input table reflects this parameter ID, it will copy the value into the parameter value register.
   // It will then trigger the next rung to read the next parameter of data.
   // The timer is a delay to give system enough time to copy the value into the register.
   140: XIC(rd_ws_rst.9)[MOV(16#49E9,Out_hi6200.Parameter_ID) ,EQU(Inp_hi6200.Parameter_ID,16#49E9) COP(Inp_hi6200.Parameter_Value,pm_49E9,1) TON(read_delay_58,?,?) ];
   // Once timer is done, will clear bit for previous rung and turn on bit to run next rung.
   141: XIC(read_delay_58.DN)OTU(rd_ws_rst.9)OTL(rd_rtz.0);
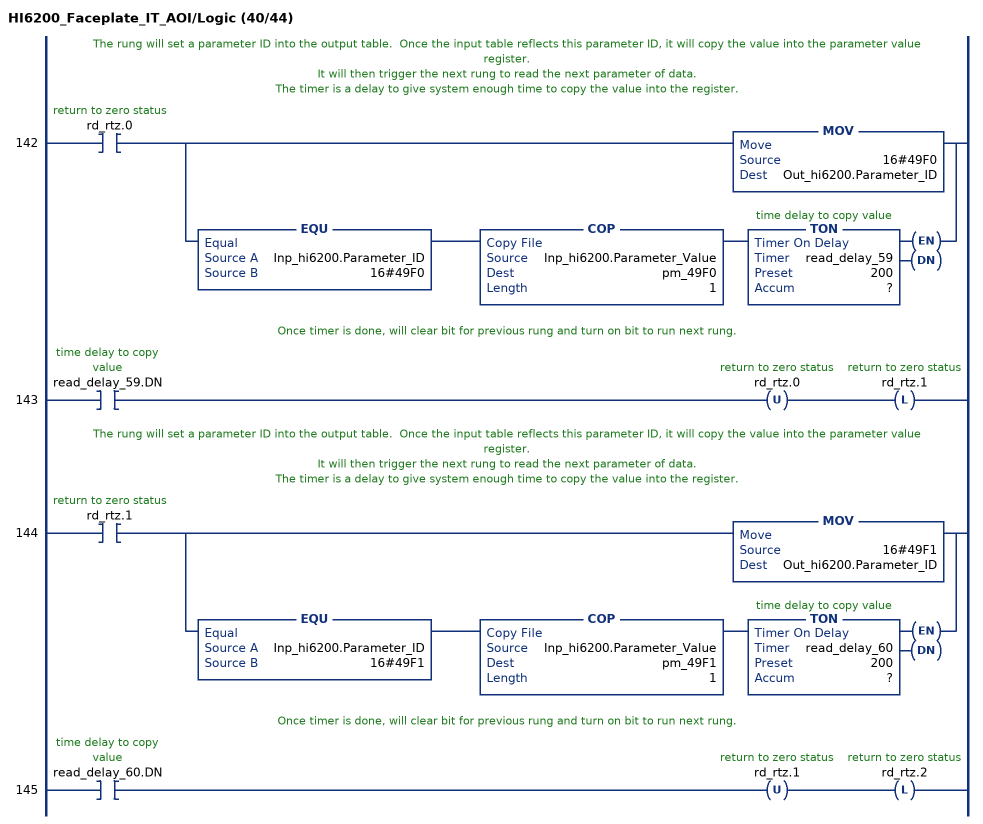
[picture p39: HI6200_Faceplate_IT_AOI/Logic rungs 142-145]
   // The rung will set a parameter ID into the output table.  Once the input table reflects this parameter ID, it will copy the value into the parameter value register.
   // It will then trigger the next rung to read the next parameter of data.
   // The timer is a delay to give system enough time to copy the value into the register.
   142: XIC(rd_rtz.0)[MOV(16#49F0,Out_hi6200.Parameter_ID) ,EQU(Inp_hi6200.Parameter_ID,16#49F0) COP(Inp_hi6200.Parameter_Value,pm_49F0,1) TON(read_delay_59,?,?) ];
   // Once timer is done, will clear bit for previous rung and turn on bit to run next rung.
   143: XIC(read_delay_59.DN)OTU(rd_rtz.0)OTL(rd_rtz.1);
   // The rung will set a parameter ID into the output table.  Once the input table reflects this parameter ID, it will copy the value into the parameter value register.
   // It will then trigger the next rung to read the next parameter of data.
   // The timer is a delay to give system enough time to copy the value into the register.
   144: XIC(rd_rtz.1)[MOV(16#49F1,Out_hi6200.Parameter_ID) ,EQU(Inp_hi6200.Parameter_ID,16#49F1) COP(Inp_hi6200.Parameter_Value,pm_49F1,1) TON(read_delay_60,?,?) ];
   // Once timer is done, will clear bit for previous rung and turn on bit to run next rung.
   145: XIC(read_delay_60.DN)OTU(rd_rtz.1)OTL(rd_rtz.2);
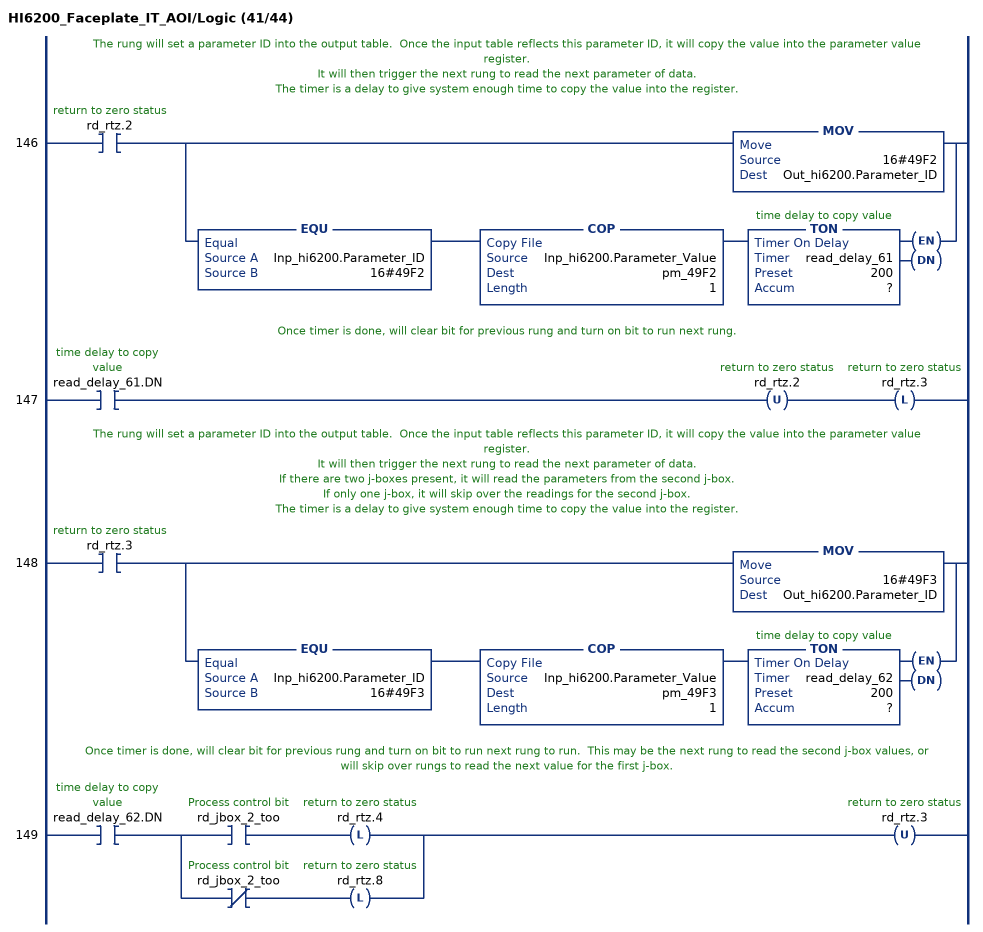
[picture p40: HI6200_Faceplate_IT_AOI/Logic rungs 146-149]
   // The rung will set a parameter ID into the output table.  Once the input table reflects this parameter ID, it will copy the value into the parameter value register.
   // It will then trigger the next rung to read the next parameter of data.
   // The timer is a delay to give system enough time to copy the value into the register.
   146: XIC(rd_rtz.2)[MOV(16#49F2,Out_hi6200.Parameter_ID) ,EQU(Inp_hi6200.Parameter_ID,16#49F2) COP(Inp_hi6200.Parameter_Value,pm_49F2,1) TON(read_delay_61,?,?) ];
   // Once timer is done, will clear bit for previous rung and turn on bit to run next rung.
   147: XIC(read_delay_61.DN)OTU(rd_rtz.2)OTL(rd_rtz.3);
   // The rung will set a parameter ID into the output table.  Once the input table reflects this parameter ID, it will copy the value into the parameter value register.
   // It will then trigger the next rung to read the next parameter of data.
   // If there are two j-boxes present, it will read the parameters from the second j-box.
   // If only one j-box, it will skip over the readings for the second j-box.
   // The timer is a delay to give system enough time to copy the value into the register.
   148: XIC(rd_rtz.3)[MOV(16#49F3,Out_hi6200.Parameter_ID) ,EQU(Inp_hi6200.Parameter_ID,16#49F3) COP(Inp_hi6200.Parameter_Value,pm_49F3,1) TON(read_delay_62,?,?) ];
   // Once timer is done, will clear bit for previous rung and turn on bit to run next rung to run.  This may be the next rung to read the second j-box values, or will skip over rungs to read the next value for the first j-box.
   149: XIC(read_delay_62.DN)[XIC(rd_jbox_2_too) OTL(rd_rtz.4) ,XIO(rd_jbox_2_too) OTL(rd_rtz.8) ]OTU(rd_rtz.3);
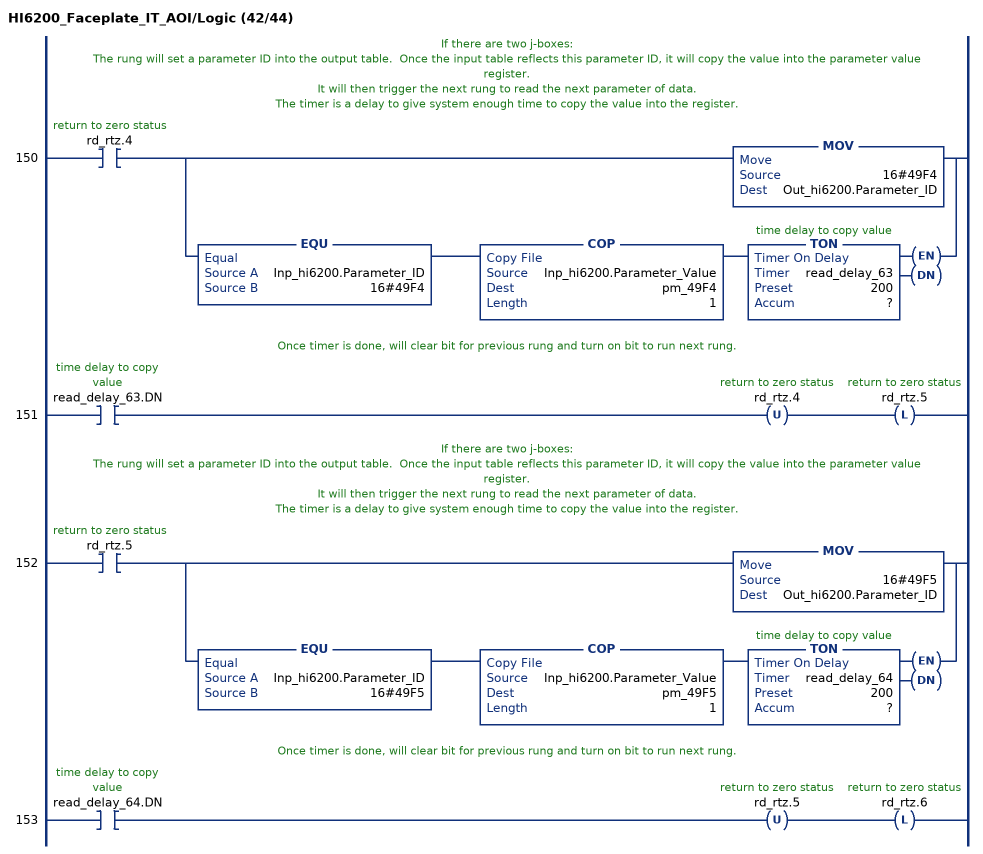
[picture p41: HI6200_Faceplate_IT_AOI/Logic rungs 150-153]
   // If there are two j-boxes:
   // The rung will set a parameter ID into the output table.  Once the input table reflects this parameter ID, it will copy the value into the parameter value register.
   // It will then trigger the next rung to read the next parameter of data.
   // The timer is a delay to give system enough time to copy the value into the register.
   150: XIC(rd_rtz.4)[MOV(16#49F4,Out_hi6200.Parameter_ID) ,EQU(Inp_hi6200.Parameter_ID,16#49F4) COP(Inp_hi6200.Parameter_Value,pm_49F4,1) TON(read_delay_63,?,?) ];
   // Once timer is done, will clear bit for previous rung and turn on bit to run next rung.
   151: XIC(read_delay_63.DN)OTU(rd_rtz.4)OTL(rd_rtz.5);
   // If there are two j-boxes:
   // The rung will set a parameter ID into the output table.  Once the input table reflects this parameter ID, it will copy the value into the parameter value register.
   // It will then trigger the next rung to read the next parameter of data.
   // The timer is a delay to give system enough time to copy the value into the register.
   152: XIC(rd_rtz.5)[MOV(16#49F5,Out_hi6200.Parameter_ID) ,EQU(Inp_hi6200.Parameter_ID,16#49F5) COP(Inp_hi6200.Parameter_Value,pm_49F5,1) TON(read_delay_64,?,?) ];
   // Once timer is done, will clear bit for previous rung and turn on bit to run next rung.
   153: XIC(read_delay_64.DN)OTU(rd_rtz.5)OTL(rd_rtz.6);
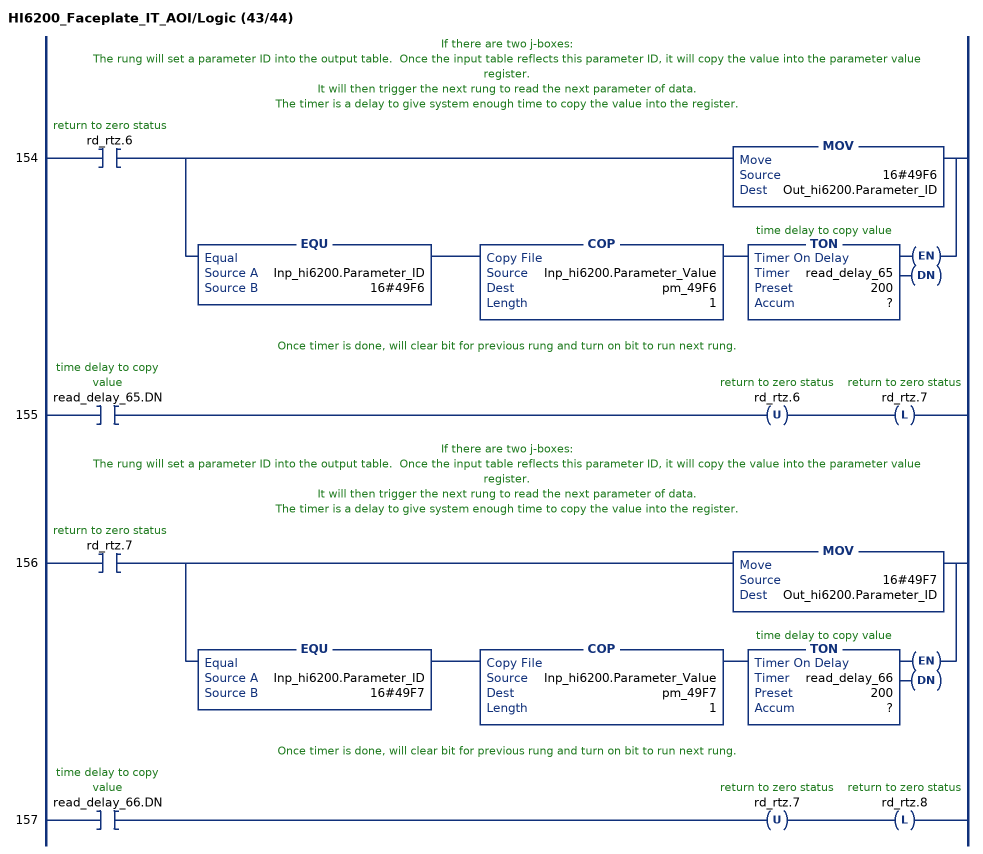
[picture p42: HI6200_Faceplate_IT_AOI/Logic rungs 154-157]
   // If there are two j-boxes:
   // The rung will set a parameter ID into the output table.  Once the input table reflects this parameter ID, it will copy the value into the parameter value register.
   // It will then trigger the next rung to read the next parameter of data.
   // The timer is a delay to give system enough time to copy the value into the register.
   154: XIC(rd_rtz.6)[MOV(16#49F6,Out_hi6200.Parameter_ID) ,EQU(Inp_hi6200.Parameter_ID,16#49F6) COP(Inp_hi6200.Parameter_Value,pm_49F6,1) TON(read_delay_65,?,?) ];
   // Once timer is done, will clear bit for previous rung and turn on bit to run next rung.
   155: XIC(read_delay_65.DN)OTU(rd_rtz.6)OTL(rd_rtz.7);
   // If there are two j-boxes:
   // The rung will set a parameter ID into the output table.  Once the input table reflects this parameter ID, it will copy the value into the parameter value register.
   // It will then trigger the next rung to read the next parameter of data.
   // The timer is a delay to give system enough time to copy the value into the register.
   156: XIC(rd_rtz.7)[MOV(16#49F7,Out_hi6200.Parameter_ID) ,EQU(Inp_hi6200.Parameter_ID,16#49F7) COP(Inp_hi6200.Parameter_Value,pm_49F7,1) TON(read_delay_66,?,?) ];
   // Once timer is done, will clear bit for previous rung and turn on bit to run next rung.
   157: XIC(read_delay_66.DN)OTU(rd_rtz.7)OTL(rd_rtz.8);
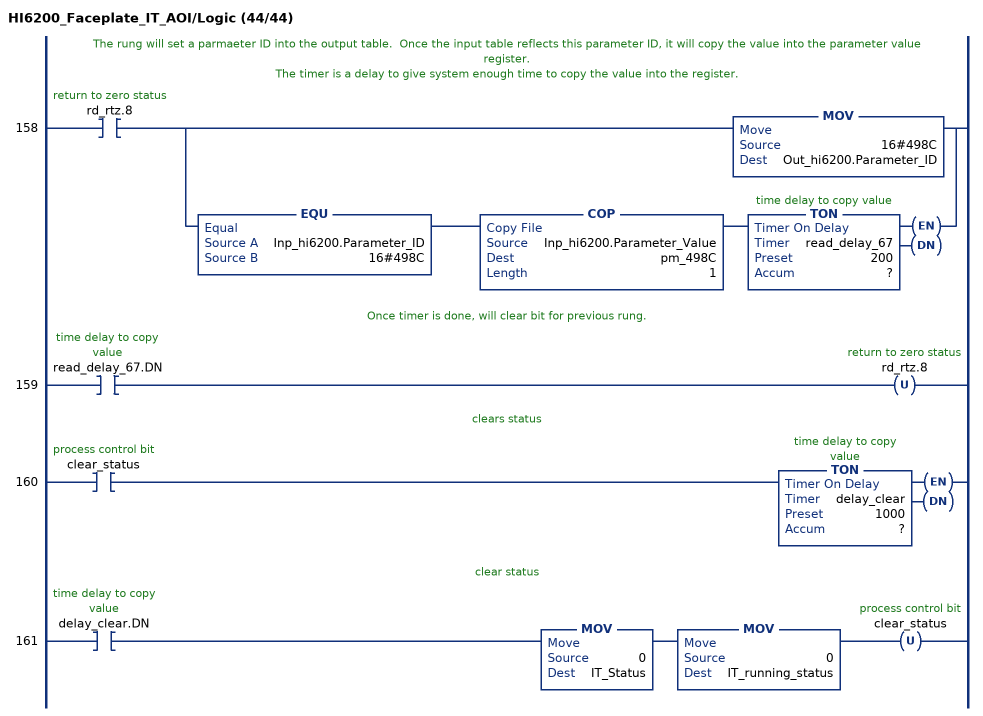
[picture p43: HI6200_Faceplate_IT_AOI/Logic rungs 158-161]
   // The rung will set a parmaeter ID into the output table.  Once the input table reflects this parameter ID, it will copy the value into the parameter value register.
   // The timer is a delay to give system enough time to copy the value into the register.
   158: XIC(rd_rtz.8)[MOV(16#498C,Out_hi6200.Parameter_ID) ,EQU(Inp_hi6200.Parameter_ID,16#498C) COP(Inp_hi6200.Parameter_Value,pm_498C,1) TON(read_delay_67,?,?) ];
   // Once timer is done, will clear bit for previous rung.
   159: XIC(read_delay_67.DN)OTU(rd_rtz.8);
   // clears status
   160: XIC(clear_status)TON(delay_clear,?,?);
   // clear status
   161: XIC(delay_clear.DN)MOV(0,IT_Status)MOV(0,IT_running_status)OTU(clear_status);
END_ROUTINE
END_ADD_ON_INSTRUCTION
